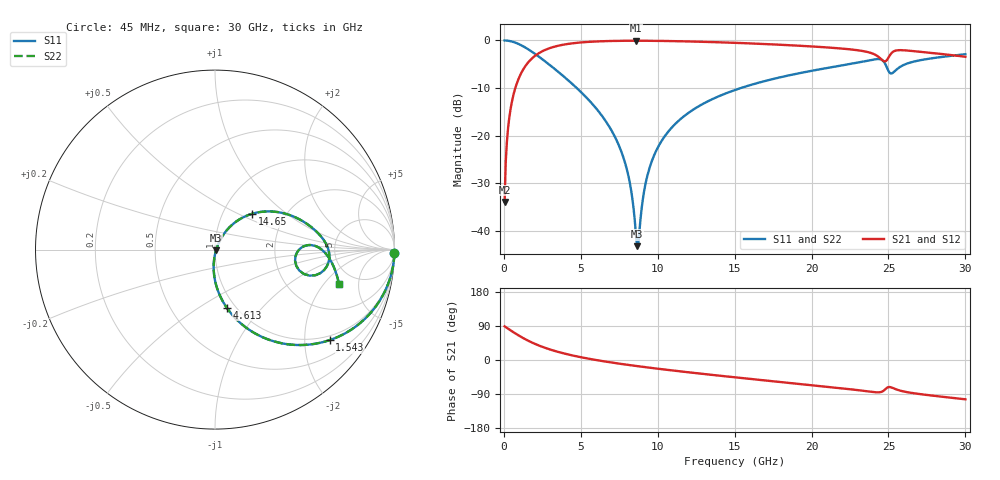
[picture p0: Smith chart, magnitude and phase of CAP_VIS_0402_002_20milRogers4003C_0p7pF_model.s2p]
! S-parameter model data by Modelithics Inc.  support@modelithics.com  813-866-6335  Tampa FL USA
! S-Parameter data specifications:
! Substrate: 20-mil Rogers 4003C, substrate thickness, H=0.508mm, Dielectric constant, Er=3.75
! PCB Mounting Pad Footprint: Pad width, PadW=0.50mm , Pad length, PadL=0.50mm , Pad gap, PadG (edge-to-edge)=0.40mm , Reference planes=1.4mm apart
! Created Wed Nov 18 12:39:53 2015
# hz S ma R 50
! 2 Port Network Data from SP1.SP block
! freq  magS11  angS11  magS21  angS21  magS12  angS12  magS22  angS22
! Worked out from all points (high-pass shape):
!   401 points, 45 MHz to 30 GHz, reference 50 ohm
!   highest |S21| = -0.06 dB at 8.582 GHz (marker M1); lowest = -33.9 dB at 45 MHz (marker M2)
!   |S21| within 3 dB of the highest: 2.095 GHz to 24.17 GHz (22.08 GHz wide, 168 % of centre); 25.1 GHz to 29.05 GHz (3.945 GHz wide, 14.6 % of centre)
!   lowest |S11| = -43.2 dB at 8.657 GHz (marker M3), VSWR 1.01, Z = 50.6 - j0.371 ohm
!   |S11| at or under -10 dB: 4.735 GHz to 15.4 GHz (10.67 GHz wide, 106 % of centre)
!   |S22| runs from -43.2 to 0.0 dB; largest |S21 - S12| = 0
!   S11 on the Smith chart (normalised r, x): 45 MHz: 1, -93; 1.543 GHz: 0.88, -2.62; 4.613 GHz: 0.91, -0.66; 14.65 GHz: 1.37, +0.60; 30 GHz: 3.67, -2.89
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4.5e7  0.9998 -1.2  0.0201 88.8  0.0201 88.8  0.9998 -1.2
2.696625e8  0.9928 -7.4  0.1197 82.6  0.1197 82.6  0.9928 -7.4
4.94325e8  0.9762 -13.4  0.2163 76.6  0.2163 76.6  0.9762 -13.4
1.54275e9  0.8142 -38.3  0.5789 51.6  0.5789 51.6  0.8142 -38.3
2.965612e9  0.5545 -61.6  0.8289 28.1  0.8289 28.1  0.5545 -61.6
4.613138e9  0.3298 -78.6  0.9394 10.6  0.9394 10.6  0.3298 -78.6
5.062462e9  0.2814 -82.2  0.9547 6.9  0.9547 6.9  0.2814 -82.2
7.53375e9  0.07474 -95.1  0.9909 -9.8  0.9909 -9.8  0.07474 -95.1
8.13285e9  0.03519 -92.8  0.9928 -13.2  0.9928 -13.2  0.03519 -92.8
8.582175e9  0.00923 -60.1  0.9931 -15.7  0.9931 -15.7  0.00923 -60.1
8.657062e9  0.006892 -32.1  0.9931 -16.1  0.9931 -16.1  0.006892 -32.1
8.806838e9  0.009756 29.8  0.993 -16.9  0.993 -16.9  0.009756 29.8
9.33105e9  0.03821 60.0  0.9921 -19.6  0.9921 -19.6  0.03821 60.0
1.007992e10  0.07895 61.4  0.9894 -23.4  0.9894 -23.4  0.07895 61.4
1.180234e10  0.1644 55.7  0.9782 -31.6  0.9782 -31.6  0.1644 55.7
1.464806e10  0.2867 44.1  0.9487 -44.1  0.9487 -44.1  0.2867 44.1
1.50225e10  0.3015 42.5  0.944 -45.7  0.944 -45.7  0.3015 42.5
2.003996e10  0.481 22.1  0.8645 -66.6  0.8645 -66.6  0.481 22.1
2.423366e10  0.6374 -2.5  0.6939 -85.3  0.6939 -85.3  0.6374 -2.5
2.505742e10  0.4613 -11.2  0.6853 -71.3  0.6853 -71.3  0.4613 -11.2
2.595608e10  0.5498 2.4  0.7891 -82.8  0.7891 -82.8  0.5498 2.4
3e10  0.7165 -15.5  0.6733 -103.7  0.6733 -103.7  0.7165 -15.5
